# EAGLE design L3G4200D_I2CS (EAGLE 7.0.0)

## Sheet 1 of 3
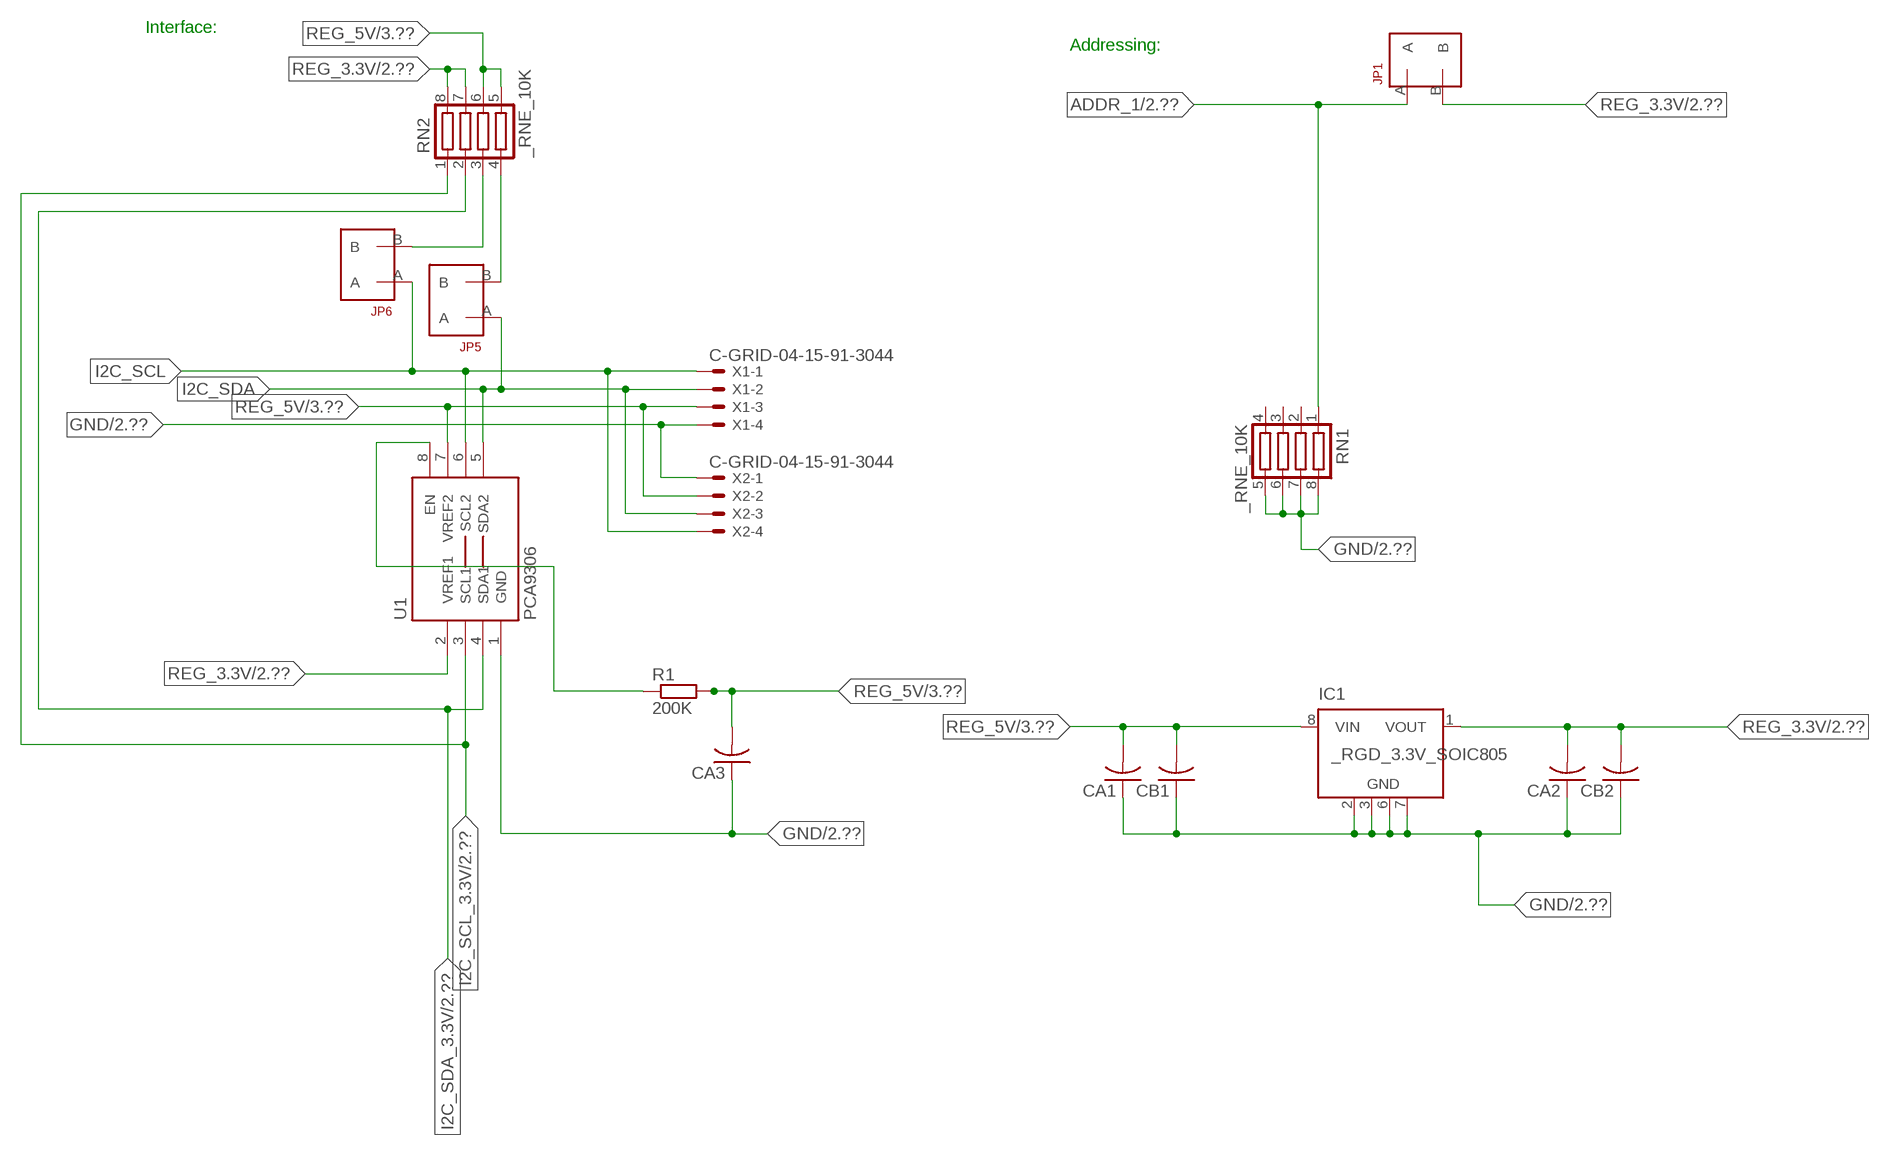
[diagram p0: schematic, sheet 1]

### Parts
CA1  CC1206KRX7R9BB104  [.1UF]
CA2  CC1206KRX7R9BB104  [.1UF]
CA3  CC1206KRX7R9BB104  [.1UF]
CB1  TMK316F106ZL-TC1206K  [TMK316F106ZL-T]
CB2  TMK316F106ZL-TC1206K  [TMK316F106ZL-T]
IC1  _RGD_3.3V_SOIC805  [_RGC_3.3V_SOIC8]
JP1  JUMPER_1X2_2MM  [JUMPER_1X2_2MM]
JP5  JUMPER_1X2_2MM  [JUMPER_1X2_2MM]
JP6  JUMPER_1X2_2MM  [JUMPER_1X2_2MM]
R1  200K  RESISTOR_SMT-0603  [R603]
RN1  _RNE_10K  [RNE]
RN2  _RNE_10K  [RNE]
U1  PCA9306  PCA9306_NCD  [PSOP-8]
X1  C-GRID-04-15-91-3044  [15-91-04]
X2  C-GRID-04-15-91-3044  [15-91-04]

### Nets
ADDR_1: JP1.A RN1.1 ; also sheet 2
GND: CA1.1 CA2.1 CA3.1 CB1.1 CB2.1 IC1.2(GND) IC1.3(GND) IC1.6(GND) IC1.7(GND) RN1.5 RN1.6 RN1.7 RN1.8 U1.1(GND) X1.4 X2.1 ; also sheet 2,3
I2C_SCL: JP6.A U1.6(SCL2) X1.1 X2.4
I2C_SCL_3.3V: RN2.1 U1.3(SCL1) ; also sheet 2
I2C_SDA: JP5.A U1.5(SDA2) X1.2 X2.3
I2C_SDA_3.3V: RN2.2 U1.4(SDA1) ; also sheet 2
N$1: JP6.B RN2.3
N$2: JP5.B RN2.4
N$3: R1.1 U1.8(EN)
REG_3.3V: CA2.2 CB2.2 IC1.1(VOUT) JP1.B RN2.7 RN2.8 U1.2(VREF1) ; also sheet 2
REG_5V: CA1.2 CA3.2 CB1.2 IC1.8(VIN) R1.2 RN2.5 RN2.6 U1.7(VREF2) X1.3 X2.2 ; also sheet 3
Unconnected: IC1.4(NC) IC1.5(NC) RN1.2 RN1.3 RN1.4

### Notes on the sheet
- Interface:
- Addressing:

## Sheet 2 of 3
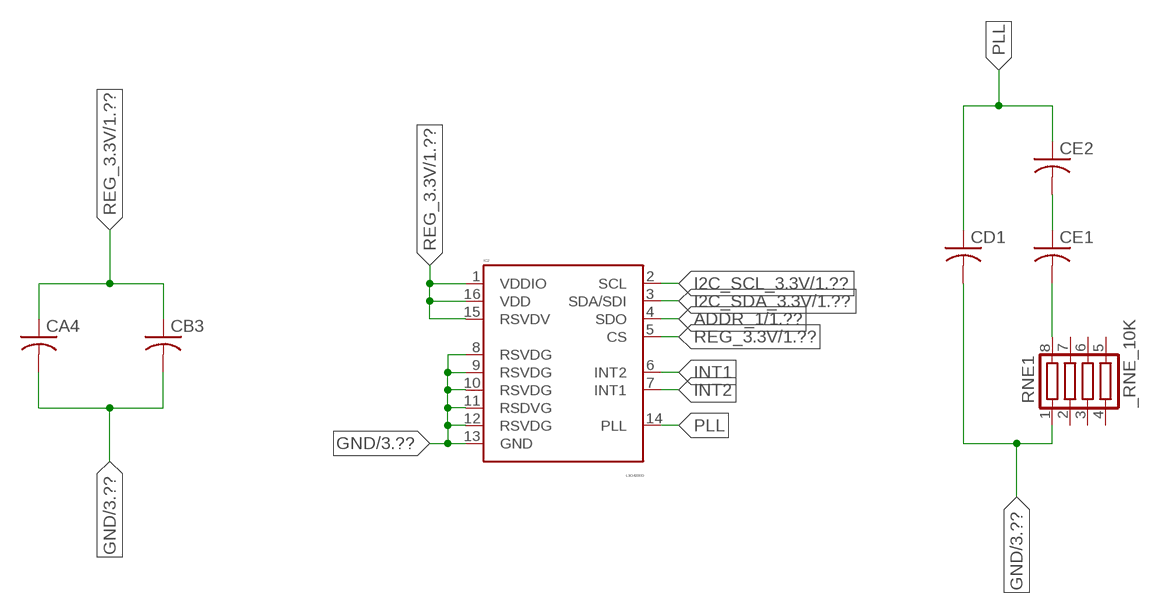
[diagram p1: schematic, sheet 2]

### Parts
CA4  _CA_.10UF_50VC1206K  [_CA_.1UF_50V]
CB3  _CB_10UF_25VC1206K  [_CB_10UF_25V]
CD1  _CD_10NF_50VC1206K  [_CD_10NF_50V]
CE1  CC0603JRNPO8BN1020603  [CC0603JRNPO8BN102]
CE2  CC0603JRNPO8BN1020603  [CC0603JRNPO8BN102]
IC2  L3G4200D  [LGA16-4X4]
RNE1  _RNE_10K  [RNE]

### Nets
ADDR_1: IC2.4(SDO) ; also sheet 1
GND: CA4.2 CB3.2 CD1.2 IC2.8(RSVDG) IC2.9(RSVDG) IC2.10(RSVDG) IC2.11(RSDVG) IC2.12(RSVDG) IC2.13(GND) RNE1.1 ; also sheet 1,3
I2C_SCL_3.3V: IC2.2(SCL) ; also sheet 1
I2C_SDA_3.3V: IC2.3(SDA/SDI) ; also sheet 1
INT1: IC2.6(INT2)
INT2: IC2.7(INT1)
N$14: CE1.1 CE2.2
N$15: CE1.2 RNE1.8
PLL: CD1.1 CE2.1 IC2.14(PLL)
REG_3.3V: CA4.1 CB3.1 IC2.1(VDDIO) IC2.5(CS) IC2.15(RSVDV) IC2.16(VDD) ; also sheet 1
Unconnected: RNE1.2 RNE1.3 RNE1.4 RNE1.5 RNE1.6 RNE1.7

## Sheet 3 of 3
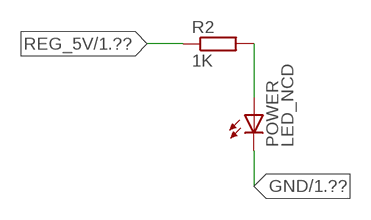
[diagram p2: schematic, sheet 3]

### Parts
POWER  LED_NCD  [CHIPLED_0603]
R2  1K  RESISTOR_SMT-0402  [R402]

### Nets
GND: POWER.C ; also sheet 1,2
N$4: POWER.A R2.2
REG_5V: R2.1 ; also sheet 1

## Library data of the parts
CA1-CA3 = NCD_ULTIMATE_LIBRARY:CC1206KRX7R9BB104: Capacitor CA .1uF 50V SMT C1206K CC1206KRX7R9BB104
CA4 = NCD_ULTIMATE_LIBRARY (2):_CA_.10UF_50V: Capacitor .1uF SMT
CB1 CB2 = NCD_ULTIMATE_LIBRARY:TMK316F106ZL-T: Capacitor CB 10uF SMT 1206 TMK316F106ZL-T
CB3 = NCD_ULTIMATE_LIBRARY (2):_CB_10UF_25V: Capacitor 10uF SMT
CD1 = NCD_ULTIMATE_LIBRARY (2):_CD_10NF_50V: Capacitor 10nF SMT
CE1 CE2 = NCD_ULTIMATE_LIBRARY (2):CC0603JRNPO8BN102: Capacitor CE 1uF SMT CC0603JRNPO8BN102 0603
IC1 = NCD_ULTIMATE_LIBRARY:_RGD_3.3V_SOIC8: Regulator Linear 3.3V Chip Positive VOLTAGE REGULATOR Digikey 497-1199-2-ND/L78L33ACD13TR
IC2 = NCD_ULTIMATE_KAMNA:L3G4200D: L3G4200D Three-axis, digital output gyroscope The L3G4200D is a low-power three-axis angular rate sensor, has a full scale of ±250/±500/±2000 dps and is capable of measuring rates with a user-selectable bandwidth. It includes a sensing element and an IC interface capable of providing the measured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
JP1 JP5 JP6 = NCD_ULTIMATE_CONNECTORS:JUMPER_1X2_2MM
POWER = NCD_ULTIMATE_LIBRARY:LED_NCD: LED Digikey 754-1132-2-ND/APT2012SRCPRV
R1 R2 = NCD_ULTIMATE_LIBRARY:RESISTOR_SMT: NCD Resistor
RN1 RN2 = NCD_ULTIMATE_LIBRARY:_RNE_10K: Resistor Array RNE SMT 10K x 4 Single Resistor Source: http://www.ctscorp.com/components/Datasheets/CTSChipArrayDs.pdf Digikey 742C083103JPTR-ND/742C083103JP; OC_FARNELL: unknown; OC_NEWARK: unknown
RNE1 = NCD_ULTIMATE_LIBRARY (2):_RNE_10K: Resistor Array RNE SMT 10K x 4 Single Resistor Source: http://www.ctscorp.com/components/Datasheets/CTSChipArrayDs.pdf Digikey 742C083103JPTR-ND/742C083103JP; OC_FARNELL: unknown; OC_NEWARK: unknown
U1 = NCD_ULTIMATE_LIBRARY:PCA9306_NCD: NCD Bidirectional I2C level shifter. NOT compatible with all available part number pinout schemes- DOUBLE CHECK!!!; PROD_ID: IC-10023
X1 X2 = NCD_ULTIMATE_CONNECTORS:C-GRID-04: CONNECTOR 4-Pos I2C wire to board 2.54 mm (0.100") pitch header Digikey WM1342-ND/0015912045; OC_FARNELL: unknown; OC_NEWARK: unknown

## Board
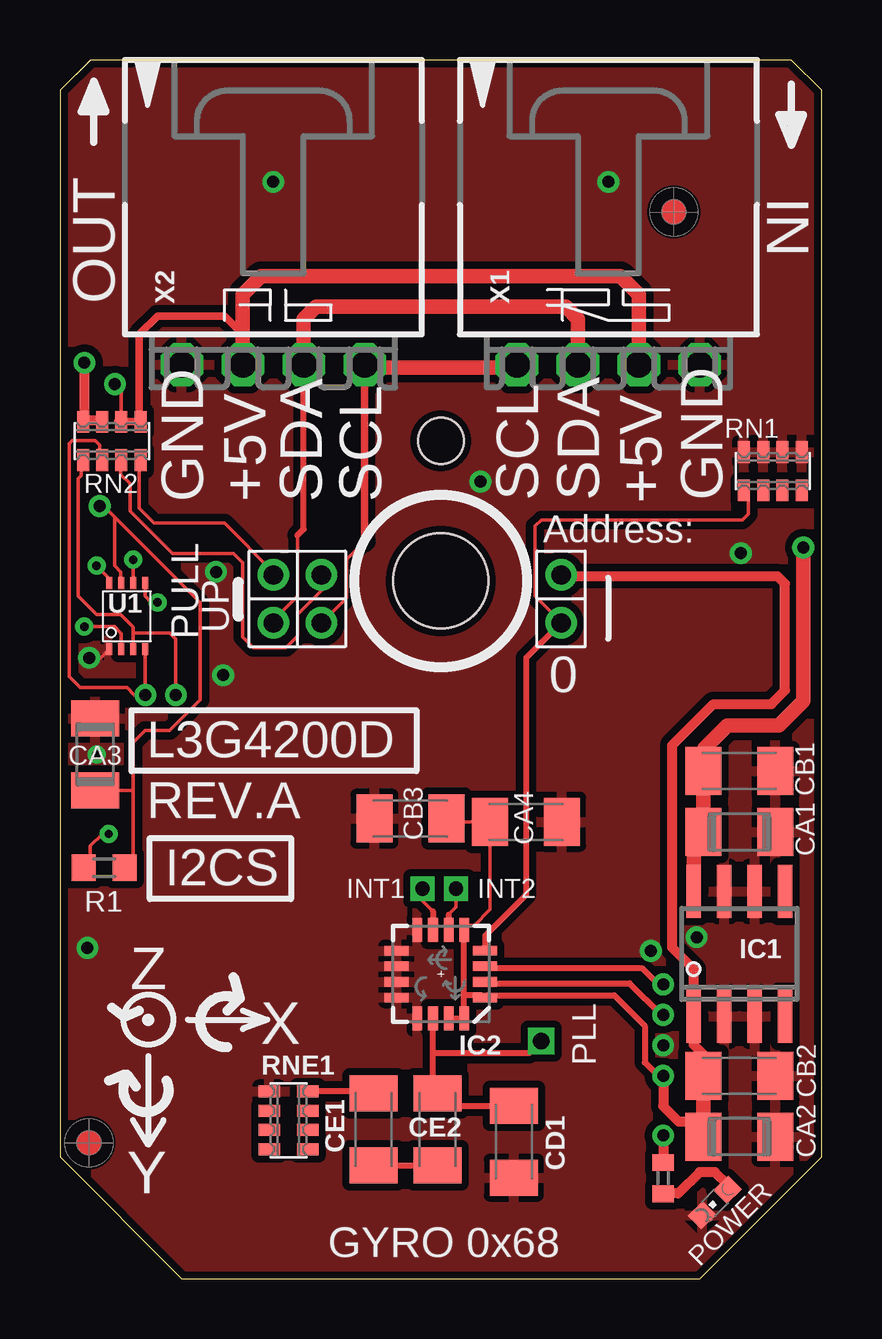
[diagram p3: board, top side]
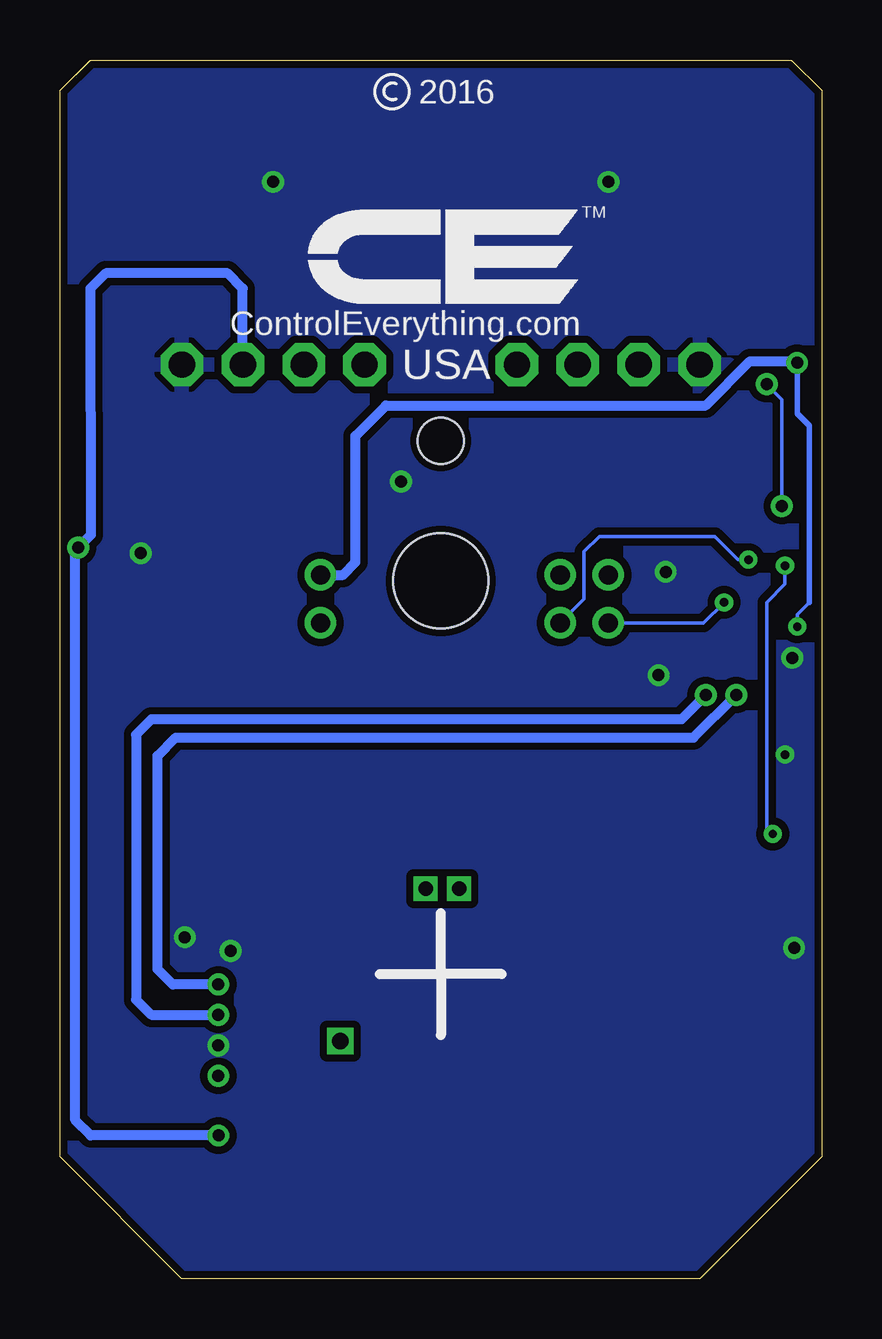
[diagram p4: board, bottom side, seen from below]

Size 31.75 x 50.8 mm. Coordinates in mm from the lower left corner, seen from the top.
Outline: 32 segments
Copper layers (1*16): Top 0.035mm / dielectric 1.5mm / Bottom 0.035mm
Design rules "default": minimum track width 5mil, minimum drill 24mil, track to track 5mil, track to pad 5mil, pad to pad 5mil, via to via 5mil, smd to smd 5mil, copper to edge 10mil, drill to drill 8mil, minimum pad ring 10mil, minimum via ring 8mil, stop-mask expansion 2mil, vias tented up to drill 0mil, thermal gap 10mil
Holes 3.96 mm at 15.88,29.08
Holes 1.91 mm at 15.88,34.93

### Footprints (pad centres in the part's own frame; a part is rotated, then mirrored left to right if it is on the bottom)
.1UF = smd 1.5 x 2: 1 -1.5,0; 2 1.5,0
_CA_.1UF_50V = smd 1.5 x 2: 1 -1.5,0; 2 1.5,0
TMK316F106ZL-T = smd 1.5 x 2: 1 -1.5,0; 2 1.5,0
_CB_10UF_25V = smd 1.5 x 2: 1 -1.5,0; 2 1.5,0
_CD_10NF_50V = smd 1.5 x 2: 1 -1.5,0; 2 1.5,0
CC0603JRNPO8BN102 = smd 1.5 x 2: 1 -1.5,0; 2 1.5,0
_RGC_3.3V_SOIC8 = smd 0.6 x 2.2: 1 -1.905,-2.6; 2 -0.635,-2.6; 3 0.635,-2.6; 4 1.905,-2.6; 5 1.905,2.6; 6 0.635,2.6; 7 -0.635,2.6; 8 -1.905,2.6
LGA16-4X4 = smd 1 x 0.4: 1 -1.85,0.975; 2 -1.85,0.325; 3 -1.85,-0.325; 4 -1.85,-0.975; 9 1.85,-0.975; 10 1.85,-0.325; 11 1.85,0.325; 12 1.85,0.975 | smd 0.4 x 1: 5 -0.975,-1.85; 6 -0.325,-1.85; 7 0.325,-1.85; 8 0.975,-1.85; 13 0.975,1.85; 14 0.325,1.85; 15 -0.325,1.85; 16 -0.975,1.85
JUMPER_1X2_2MM = drill 0.8: A 0,2; B 0,0
CHIPLED_0603 = smd 0.8 x 0.876: A 0,-0.75; C 0,0.75
R603 = smd 1 x 1.1: 1 -0.85,0; 2 0.85,0
R402 = smd 0.7 x 0.9: 1 -0.65,0; 2 0.65,0
RNE = smd 0.5 x 0.9: 1 -1.2,-0.8; 2 -0.4,-0.8; 3 0.4,-0.8; 4 1.2,-0.8; 5 1.2,0.8; 6 0.4,0.8; 7 -0.4,0.8; 8 -1.2,0.8
PSOP-8 = smd 0.25 x 0.5: 1 -0.73,-1.37; 2 -0.23,-1.37; 3 0.27,-1.37; 4 0.77,-1.37; 5 0.77,1.38; 6 0.27,1.38; 7 -0.23,1.38; 8 -0.73,1.38
15-91-04 = drill 1.1 pad 1.778 octagon: 1 -3.81,-7.62; 2 -1.27,-7.62; 3 1.27,-7.62; 4 3.81,-7.62

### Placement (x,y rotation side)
CA1  28.32,18.62 180 top
CA2  28.32,5.92 180 top
CA3  1.46,21.86 270 top
CA4  19.43,19.05 0 top
CB1  28.32,21.16 180 top
CB2  28.32,8.46 180 top
CB3  14.61,19.18 180 top
CD1  18.92,5.72 270 top
CE1  13.08,6.22 90 top
CE2  15.75,6.22 270 top
IC1  28.32,13.54 0 top
IC2  15.88,12.7 180 top
JP1  20.89,29.34 180 top
JP5  8.89,29.34 180 top
JP6  10.9,29.34 180 top
POWER  27.3,3.18 135 top
R1  1.84,17.13 0 top
R2  25.15,4.19 270 top
RN1  29.72,33.66 0 top
RN2  2.16,34.93 0 top
RNE1  9.53,6.6 270 top
U1  2.79,27.61 0 top
U$5  [VISION_REF10]  1.21,5.66 90 top
U$28  [VISION_REF10]  25.59,44.46 90 top
X1  22.86,45.72 0 top
X2  8.89,45.72 0 top

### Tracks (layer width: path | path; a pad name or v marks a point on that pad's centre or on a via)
ADDR_1
  Top 0.152: JP1.A 20.89,27.37 19.81,28.45 19.81,31.37 20.07,31.62 28.45,31.62 28.7,31.88 28.7,32.78 RN1.1
  Top 0.254: JP1.A 19.43,25.87 19.43,16 17.73,14.3 IC2.4
GND  (via drill 0.35, 0.5)
  Top 0.152: CA3.1 1.52,23.42 1.52,23.62 | U1.1 1.7,25.88 v1.22,25.88
  other vias: 8.89,45.72 22.86,45.72 25.15,9.73 6.8,25.16 17.53,33.22 26.55,14.24 1.15,13.79 6.5,29.46 1.52,21.84 24.64,13.67 28.39,30.24
  pour Top (isolate 0.305): -1.27,0 -1.27,50.8 33.02,50.8 33.02,0
  pour Bottom (isolate 0.305): -5.08,0 -5.08,50.8 35.56,50.8 35.56,0
I2C_SCL  (via drill 0.35)
  Top 0.152: 12.7,30.73 11.94,29.97 11.94,28.38 JP6.A | v3.05,29.97 3.06,29.96 U1.6
  Top 0.305: 12.7,30.73 X2.4
  Top 0.406: X2.4 12.7,37.97 | 19.05,37.97 X1.1
  Top 0.61: 12.7,37.97 19.05,37.97
  Bottom 0.152: JP6.A 9.91,28.33 9.91,30.3 9.27,30.94 4.45,30.94 3.48,29.97 v3.05,29.97
I2C_SCL_3.3V  (via drill 0.5)
  Top 0.152: RN2.1 0.89,34.07 0.89,33.48 0.77,33.35 0.77,29.1 0.76,29.09 0.76,28.45 1.52,27.69 2.54,27.69 3.06,27.17 3.06,26.92 | 3.06,26.92 U1.3 | v4.83,24.33 v4.83,24.34 4.83,26.67 4.57,26.92 3.06,26.92
  Top 0.254: IC2.2 17.78,12.32 23.75,12.32 25.07,11 v25.15,11
  Bottom 0.406: v4.83,24.33 5.84,23.32 27.94,23.32 28.58,22.68 28.58,11.63 27.94,11 v25.15,11
I2C_SDA  (via drill 0.35)
  Top 0.152: JP5.A 8.89,27.44 9.91,28.45 9.91,30.99 | U1.5 3.56,28.45 3.81,28.19 v4.06,28.19
  Top 0.254: 9.91,30.99 10.16,31.25 X2.3
  Top 0.61: X2.3 10.16,40.01 10.67,40.51 21.09,40.51 21.59,40.01 X1.2
  Bottom 0.152: v4.06,28.19 4.92,27.34 JP5.A
I2C_SDA_3.3V  (via drill 0.5)
  Top 0.152: RN2.2 1.65,34.14 1.65,34.75 1.46,34.94 0.51,34.94 0.38,34.81 0.38,26.37 0.38,26.36 0.38,25.1 0.84,24.64 2.79,24.64 3.1,24.33 v3.56,24.33 v3.56,24.34 U1.4
  Top 0.254: IC2.3 17.8,12.95 24.26,12.95 24.94,12.27 v25.15,12.27
  Bottom 0.406: v25.15,12.27 27.05,12.27 27.69,12.9 27.69,21.79 26.93,22.56 5.34,22.56 v3.56,24.33
INT1  (via drill 0.6)
  Top 0.152: 16.2,15.18 16.51,15.49 v16.51,16.26
  Top 0.254: 16.2,15.18 IC2.6
INT2  (via drill 0.6)
  Top 0.152: 15.55,15.31 15.11,15.75 v15.11,16.26
  Top 0.254: 15.55,15.31 IC2.7
N$1
  Top 0.152: JP6.B 10.92,29.31 10.92,28.7 9.91,27.69 9.91,26.8 9.42,26.31 8.06,26.31 7.62,26.75 7.62,29.84 7.24,30.23 4.7,30.23 2.92,32 2.92,33.15 2.54,33.53 2.54,34.1 RN2.3
  Top 0.305: 2.54,34.02 RN2.3
N$2
  Top 0.152: JP5.B 8.89,29.46 6.86,31.5 3.94,31.5 3.3,32.13 3.3,34.07 RN2.4
  Top 0.305: 3.37,33.88 RN2.4
N$3  (via drill 0.35)
  Top 0.152: R1.1 1.27,17.41 1.27,18.03 1.78,18.54 v2.03,18.54 | v1.52,29.72 2.06,29.18 U1.8
  Bottom 0.152: v2.03,18.54 2.29,18.8 2.29,28.19 1.52,28.96 v1.52,29.72
N$4
  Top 0.406: POWER.A 27.84,3.92 27.3,4.45 26.67,4.45 25.78,3.56 25.16,3.56 R2.2
N$14
  Top 0.254: CE1.1 CE2.2
N$15
  Top 0.254: CE1.2 12.11,7.8 RNE1.8
PLL  (via drill 0.7)
  Top 0.254: CE2.1 15.49,7.62 15.55,7.68 | 15.55,7.68 15.55,9.4 | 15.55,9.4 IC2.14 | 15.55,7.68 15.6,7.72 16.11,7.22 CD1.1 | v20.07,9.91 19.56,9.4 15.55,9.4
REG_3.3V  (via drill 0.35, 0.5)
  Top 0.152: v1.02,27.18 2.29,27.18 2.56,26.9 U1.2 | CB3.1 16.23,19.05 CA4.1 17.93,15.39 17.27,14.73 17.03,14.73 IC2.5
  Top 0.254: IC2.15 IC2.16 | IC2.16 16.91,10.8 | 25.07,8.46 v25.15,8.46 24.94,8.46 24.38,9.02 24.38,10.54 23.11,11.81 17.81,11.81 IC2.1 17.68,11.68 17.56,11.81 16.85,11.81 | IC2.16 16.85,11.81 | 16.85,11.81 IC2.5
  Top 0.406: CB2.2 26.82,9.35 26.42,9.75 26.42,10.36 | v25.15,8.46 25.15,7.19 25.78,6.55 26.82,6.55 | IC1.1 26.42,12.9 25.53,13.79 25.53,22.24 27.24,23.95 29.66,23.95 30.23,24.52 30.23,28.97 29.91,29.29 20.95,29.29 JP1.B | 26.52,5.62 CA2.2 | v1.02,38.18 1.02,35.78 | 1.02,35.78 RN2.8 | 1.02,35.78 1.71,35.78 RN2.7
  Top 0.61: CB2.2 26.82,6.55 CA2.2 | 26.42,10.36 IC1.1
  Bottom 0.152: 0.51,28.19 1.02,27.69 v1.02,27.18
  Bottom 0.229: 0.51,28.19 0.51,35.56 1.02,36.07 v1.02,38.18
  Bottom 0.406: v1.02,38.18 1.08,38.24 2.99,38.24 4.83,36.4 18.16,36.4 19.43,35.13 19.43,29.87 19.94,29.34 JP1.B
REG_5V  (via drill 0.5)
  Top 0.152: RN2.6 2.56,37.01 v2.29,37.29 | R1.2 3.05,17.49 3.05,20.36 | 3.05,20.36 3.05,22.35 3.56,22.86 4.57,22.86 5.84,24.13 5.84,28.19 2.29,31.75 | CA3.2 3.05,20.36 | 2.29,31.75 1.83,32.21 v1.65,32.21 | U1.7 2.54,29.01 2.54,29.46 2.29,29.72 2.29,31.75
  Top 0.305: 7.62,39.37 7.5,39.37 | 2.42,35.74 RN2.6 RN2.5 3.31,35.8 3.31,39.37 4.07,40.13 6.86,40.13 7.62,39.37 | X2.2 7.62,39.37
  Top 0.406: v25.15,5.97 R2.1
  Top 0.61: X2.2 7.62,41.02 8.38,41.78 23.37,41.78 24.13,41.02 X1.3 | IC1.8 26.42,18.21 CA1.2 CB1.2 26.86,21.2 26.86,22.11 27.82,23.06 29.98,23.06 30.99,24.08 v30.99,30.48
  Bottom 0.152: v1.65,32.21 1.65,36.65 v2.29,37.29
  Bottom 0.406: X1.3 24.13,41.28 24.77,41.91 29.84,41.91 30.48,41.27 30.47,31 v30.99,30.48 31.11,30.36 31.11,6.6 30.48,5.97 v25.15,5.97

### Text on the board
tNames: IN | OUT | GND | +5V | SDA | SCL | SCL | SDA | +5V | GND | Address: | PULL | UP | 0 | L3G4200D | REV.A | I2CS | INT1 | INT2 | Z | X | PLL | Y | GYRO 0x68
bNames: 2016 | TM | ControlEverything.com | USA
